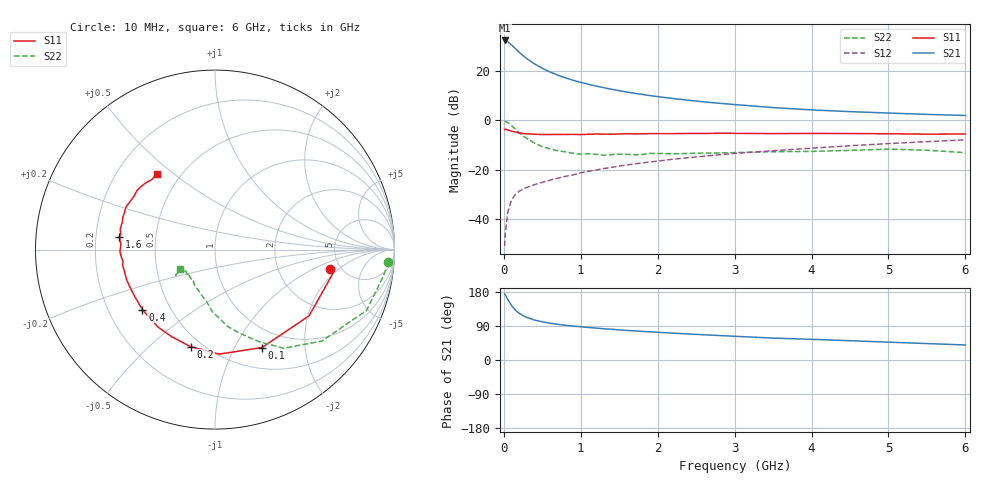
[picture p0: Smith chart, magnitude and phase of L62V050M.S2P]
!  INFINEON TECHNOLOGIES Small Signal Semiconductors
! BFR380L3 , Si-NPN RF-Transistor in TSLP-3-1
!  Vce=2 V,  Ic=50 mA
! Common Emitter S-Parameters:  07. March 2005
#  GHz  S  MA  R  50
! f  S11  S21  S12  S22
! GHz  Mag  Ang  Mag  Ang  Mag  Ang  Mag  Ang
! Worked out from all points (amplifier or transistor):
!   36 points, 10 MHz to 6 GHz, reference 50 ohm
!   highest |S21| = 32.5 dB at 10 MHz (marker M1)
!   |S21| within 3 dB of that: start of sweep to 139.8 MHz
!   unconditionally stable (mu >= 1): 1.562 GHz to 4.879 GHz
!   at 250 MHz: K = 0.48, MSG = 27.1 dB, |S12| = -27.9 dB
!   at 1.4 GHz: K = 0.99, MSG = 15.9 dB, |S12| = -19.1 dB
!   at 6 GHz: K = 0.98, MSG = 5.0 dB, |S12| = -7.9 dB
!   S11 on the Smith chart (normalised r, x): 10 MHz: 4.09, -1.55; 100 MHz: 0.75, -1.29; 200 MHz: 0.44, -0.69; 400 MHz: 0.35, -0.32; 1.6 GHz: 0.30, +0.06; 6 GHz: 0.37, +0.44
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0.01  0.6494 -9.7  42.07 174.2  0.0028 76.3  0.9689 -4.1
0.02  0.6687 -11.8  41.67 172.0  0.0053 85.8  0.9491 -9.0
0.05  0.6412 -35.1  39.65 160.0  0.0135 75.8  0.9098 -21.9
0.1  0.6053 -64.4  34.16 143.9  0.0244 64.3  0.7842 -40.5
0.15  0.5827 -87.7  28.75 131.7  0.0313 57.4  0.6694 -55.2
0.2  0.5579 -103.9  24.18 123.2  0.0366 55.4  0.568 -64.5
0.25  0.5421 -116.4  20.7 117.1  0.0403 52.3  0.4832 -73.9
0.3  0.536 -126.2  17.87 112.3  0.0438 52.3  0.4335 -80.7
0.4  0.5249 -140.4  14.03 105.3  0.0498 53.2  0.3457 -92.5
0.5  0.5178 -149.7  11.46 100.8  0.0553 55.2  0.2937 -99.2
0.6  0.5182 -156.6  9.626 97.1  0.0612 56.2  0.265 -106.3
0.7  0.5203 -161.5  8.349 94.2  0.0674 58.6  0.243 -113.0
0.9  0.522 -170.5  6.544 89.6  0.0783 61.1  0.2156 -123.8
1.1  0.5243 -175.8  5.417 85.8  0.0927 63.0  0.211 -129.2
1.3  0.5265 178.6  4.622 82.4  0.1055 63.8  0.1969 -136.7
1.6  0.537 172.3  3.773 78.0  0.1246 64.5  0.2044 -143.4
2.2  0.539 163.2  2.788 70.8  0.1629 65.3  0.21 -145.3
2.8  0.5494 154.8  2.234 64.6  0.2004 65.1  0.2185 -150.5
3.5  0.5404 146.6  1.823 57.8  0.2429 63.0  0.2315 -148.9
4.5  0.5422 140.3  1.51 50.9  0.3064 61.1  0.247 -147.9
5.5  0.5261 132.3  1.327 43.4  0.3708 57.1  0.248 -147.5
6  0.5307 127.4  1.261 39.6  0.4033 54.8  0.2219 -150.8
